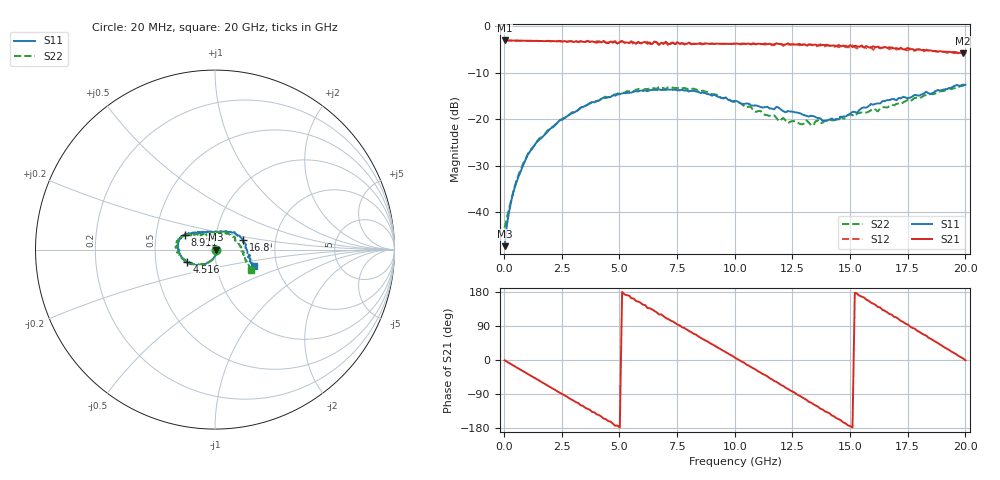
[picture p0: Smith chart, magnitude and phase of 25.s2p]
!Agilent Technologies,N5230A,US43500223,A.07.50.48
!Agilent N5230A: A.07.50.48
!Date: Saturday, September 19, 2015 12:50:10
!Correction: S11(Full 2 Port(1,2))
!S21(Full 2 Port(1,2))
!S12(Full 2 Port(1,2))
!S22(Full 2 Port(1,2))
!S2P File: Measurements: S11, S21, S12, S22:
# Hz S  dB  R 50
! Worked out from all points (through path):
!   201 points, 20 MHz to 20 GHz, reference 50 ohm
!   highest |S21| = -3.02 dB at 20 MHz (marker M1); lowest = -5.8 dB at 19.9 GHz (marker M2)
!   group delay of S21, straight-line fit = 99.6 ps
!   lowest |S11| = -47.2 dB at 20 MHz (marker M3), VSWR 1.01, Z = 50.4 - j0.0309 ohm
!   |S11| at or under -10 dB: start of sweep to end of sweep
!   |S22| runs from -43.3 to -12.5 dB; largest |S21 - S12| = 0.052
!   S11 on the Smith chart (normalised r, x): 20 MHz: 1.01, -0.00; 4.516 GHz: 0.72, -0.10; 8.911 GHz: 0.71, +0.12; 16.8 GHz: 1.36, +0.15; 20 GHz: 1.52, -0.30
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2e7  -47.24 -4.0  -3.02 -0.8  -3.02 -0.8  -43.26 4.0
4.196e8  -35.26 -64.2  -3.06 -15.3  -3.05 -15.2  -35.03 -66.0
1.019e9  -27.64 -95.3  -3.10 -36.6  -3.11 -36.7  -27.53 -92.3
2.1179e9  -21.66 -120.4  -3.16 -75.9  -3.11 -75.6  -21.51 -118.0
3.4166e9  -17.30 -141.1  -3.31 -121.2  -3.50 -122.3  -17.22 -142.8
4.5155e9  -15.23 -156.0  -3.61 -161.3  -3.41 -162.9  -15.22 -159.2
5.6144e9  -14.04 -173.5  -3.42 162.2  -3.89 160.4  -13.95 -174.3
6.7133e9  -13.52 174.0  -3.97 120.4  -3.92 120.1  -13.06 176.3
7.5125e9  -13.73 165.9  -3.37 93.9  -3.65 95.0  -13.27 169.8
8.9111e9  -14.63 153.8  -3.75 45.1  -3.79 44.3  -14.28 157.1
1.001e10  -16.00 144.6  -3.71 6.1  -3.73 5.7  -16.21 144.9
1.08092e10  -17.03 139.6  -3.61 -21.9  -3.77 -22.6  -17.99 138.9
1.19081e10  -17.48 133.3  -3.80 -61.6  -3.74 -64.4  -20.36 123.2
1.34066e10  -19.31 111.9  -3.97 -116.5  -4.05 -119.4  -21.26 97.8
1.5005e10  -18.77 62.2  -4.03 -174.4  -4.50 -172.5  -18.89 57.9
1.59041e10  -16.69 41.9  -4.59 151.6  -4.45 152.0  -18.04 34.2
1.67033e10  -15.86 22.1  -4.49 121.4  -4.94 122.3  -17.16 10.9
1.68032e10  -15.64 19.2  -4.56 119.7  -4.73 119.3  -16.87 7.6
1.75025e10  -15.45 3.6  -4.62 93.6  -5.17 92.9  -15.79 -6.1
1.83017e10  -14.03 -9.8  -5.17 64.2  -4.99 62.9  -14.76 -20.7
1.99001e10  -12.71 -23.1  -5.75 4.2  -5.80 3.1  -12.50 -28.2
2e10  -12.53 -23.2  -5.72 -0.7  -5.85 -0.6  -12.72 -29.4
